ORGANIZATION_BLOCK OB 102
BEGIN
	L		MD 0
	__ASSERT==	__ACCU 1,	0
	L		102
	T		MD 0
END_ORGANIZATION_BLOCK



ORGANIZATION_BLOCK OB 1
BEGIN
	// assert 4-accus
	__FEATURE	0
	__ASSERT==	__ACCU 1,	4


	// check that OB 102 was executed
	L		MD 0
	__ASSERT==	__ACCU 1,	102


	CALL SFC 46 // STOP CPU
END_ORGANIZATION_BLOCK
